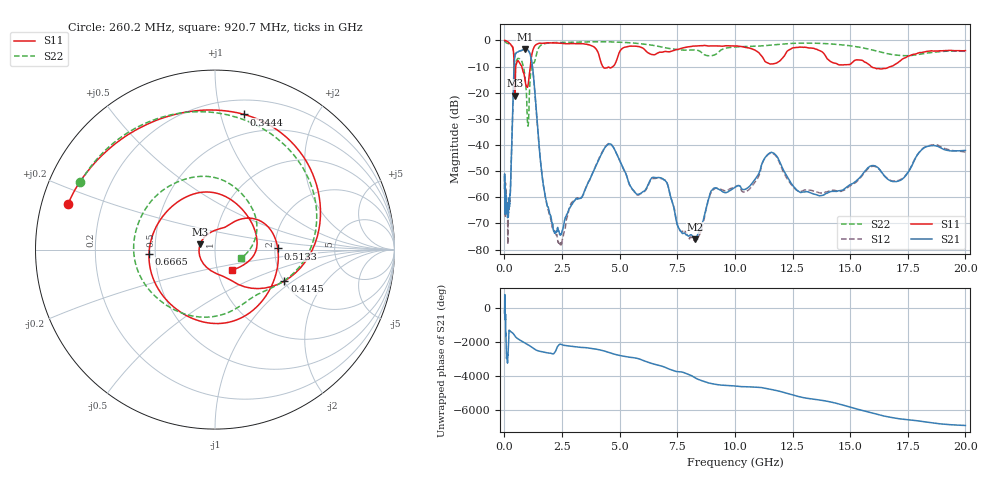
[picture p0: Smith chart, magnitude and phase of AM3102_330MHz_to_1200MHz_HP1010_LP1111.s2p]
! Date/Time: Tue, Sep 11, 2018 5:19 PM
! Network Analyzer: Agilent Technologies E8362B Rev: A.07.50.63
! Sweep from 0.010 to 20.000 GHz, 1601 Points, Sweep Type: LOG
! Power Supply: 4.949 V, 0.001 A
# Hz S DB R 50
!freq MagS11 AngS11 MagS21 AngS21 MagS12 AngS12 MagS22 AngS22
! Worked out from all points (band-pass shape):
!   1601 points, 10 MHz to 20 GHz, reference 50 ohm
!   highest |S21| = -3.26 dB at 916.3 MHz (marker M1); lowest = -76.1 dB at 8.266 GHz (marker M2)
!   |S21| within 3 dB of the highest: 449.6 MHz to 1.146 GHz (696.3 MHz wide, 87.3 % of centre)
!   lowest |S11| = -21.1 dB at 451.5 MHz (marker M3), VSWR 1.19, Z = 42.3 + j2.56 ohm
!   |S11| at or under -10 dB: 756 MHz to 1.118 GHz (361.8 MHz wide, 38.6 % of centre); 4.269 GHz to 4.705 GHz (435.8 MHz wide, 9.71 % of centre); 15.91 GHz to 16.76 GHz (845.9 MHz wide, 5.18 % of centre)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
!   |S22| runs from -32.8 to -0.2 dB; largest |S21 - S12| = 0.0091
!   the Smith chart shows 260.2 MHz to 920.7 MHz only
!   S11 on the Smith chart (normalised r, x): 260.2 MHz: 0.08, +0.15; 344.4 MHz: 0.32, +1.19; 414.5 MHz: 2.01, -0.86; 513.3 MHz: 2.08, +0.03; 666.5 MHz: 0.46, -0.02; 920.7 MHz: 1.18, -0.27
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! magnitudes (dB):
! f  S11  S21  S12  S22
! 10 MHz  0.0  -53.9  -51.7  -0.2
! 35.55 MHz  0.0  -65.1  -64.1  -0.5
! 126.4 MHz  -0.4  -63.7  -62.9  -1.1
! 146.4 MHz  -0.5  -64.7  -75.5  -1.1
! 260.2 MHz  -1.3  -58.0  -57.8  -1.5
! 344.4 MHz  -2.3  -32.2  -32.2  -2.4
! 414.5 MHz  -7.4  -11.3  -11.3  -5.8
! 447.2 MHz  -20.9  -6.4  -6.5  -9.1
! 451.5 MHz  -21.1  -6.1  -6.2  -9.3
! 513.3 MHz  -9.1  -4.7  -4.8  -8.1
! 666.5 MHz  -8.7  -4.0  -4.1  -7.1
! 916.3 MHz  -16.4  -3.3  -3.4  -15.9
! 920.7 MHz  -16.6  -3.3  -3.4  -16.3
! 1.027 GHz  -17.1  -3.8  -3.8  -32.8
! 1.59 GHz  -1.1  -48.2  -48.2  -1.8
! 2.404 GHz  -1.1  -74.3  -77.9  -0.8
! 4.479 GHz  -10.3  -40.0  -39.7  -0.5
! 5.652 GHz  -2.2  -57.9  -58.1  -1.0
! 8.266 GHz  -2.2  -76.1  -76.7  -3.6
! 11.53 GHz  -9.0  -43.0  -43.2  -1.8
! 13.81 GHz  -4.5  -59.3  -58.4  -1.2
! 20 GHz  -3.9  -42.1  -42.7  -4.2
